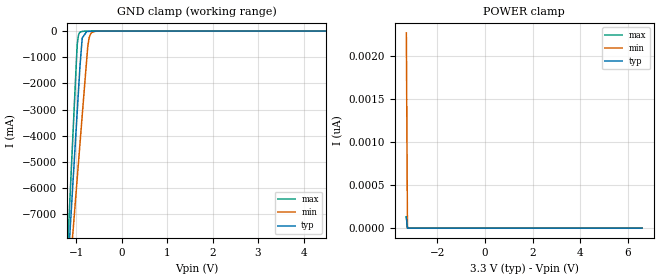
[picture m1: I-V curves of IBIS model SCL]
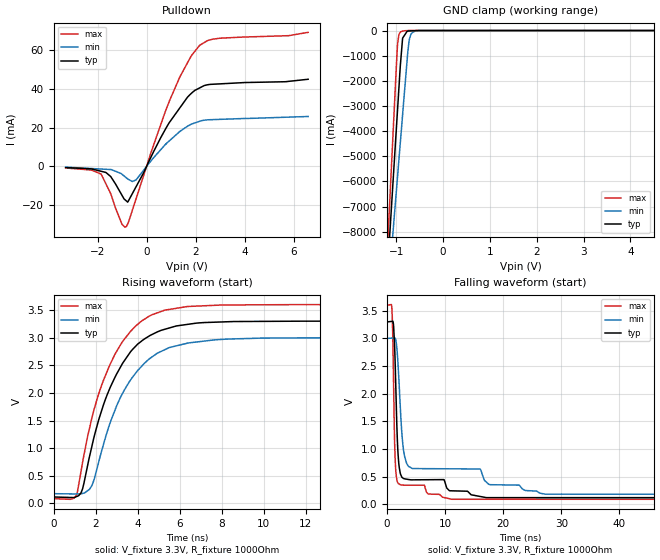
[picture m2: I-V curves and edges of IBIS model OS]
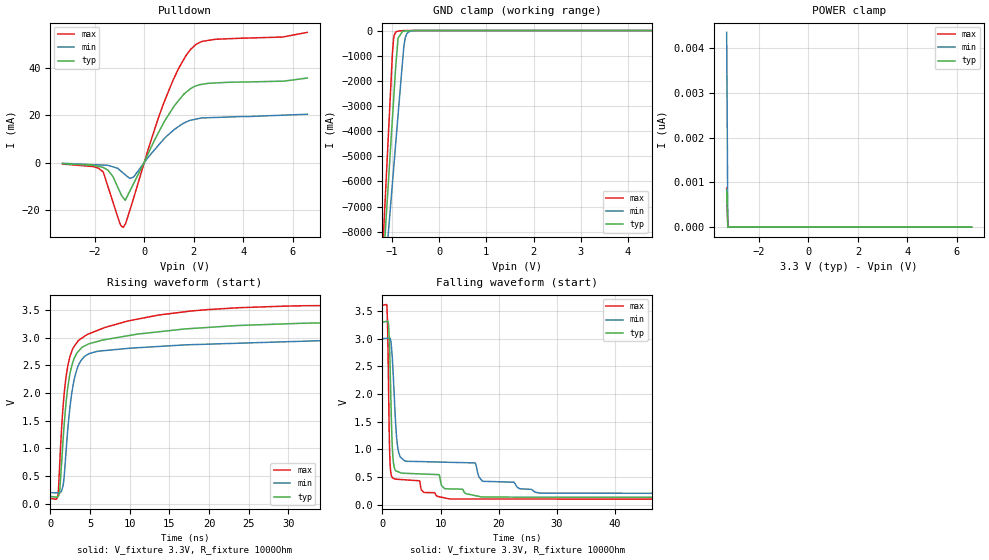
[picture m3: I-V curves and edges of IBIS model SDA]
| Texas Instruments Incorporated
| Low-Noise Clock Jitter Cleaner with Dual Loop PLLs
| Marketing part#   Voltage Range   Package-type   #pins/pkg drawing
| LM95245D   3.0V - 3.6V   SOIC   8-pin D
| LM95245DGK   3.0V - 3.6V   VSSOP   8-pin DGK
[IBIS Ver]   4.1
[File name]   lm95245.ibs
[File Rev]   1.0
[Date]   01/16/2015
[Source]   Model built from spectre simulations at:
   Texas Instruments Incorporated.
   Analog-eLab, HPA
   12500 TI Blvd
   Dallas, TX -75243
   For Support e-mail: elab_ibis@list.ti.com
[Notes]   Revision History
   Rev 1.0: 01/16/2015
   - Leakage currents at limits are high due to reverse conduction through ESD cell when reversed biased
   - Pulldown non-monotonic
   - ccomp values are based on PVT settings:
   MIN: Low Voltage, High Temperature, Weak Process
   TYP: Nominal Voltage, Nominal Temperature, Nominal Process
   MAX: High Voltage, Low Temperature, Fast Process
   - C_comp although listed in numerical order of value are obtained from varying PVT conditions.
   For PVT conditions for each specific value, refer to the buffer description under respective [Model].
   IBIS model user is responsible for using appropriate C_comp to simulate for Signal Integrity.
[Disclaimer]  This model is designed as an aid for customers of Texas Instruments
 TI and its licensors and suppliers make no warranties, either expressed
 or implied, with respect to this  model, including the warranties of
 merchantability or fitness for a particular purpose.
 The model is provided solely on an "as is" basis. The entire risk as to
 its quality and performance is with the customer.
[Copyright] (C)Copyright 2015 Texas Instruments Incorporated.
   All rights reserved.
[Component]   LM95245D
[Manufacturer]  Texas Instruments Incorporated
[Package]   |8-pin SOIC D package
|   typ   min   max
R_pkg   0.05625   0.05284   0.06331
L_pkg   2.58853nH   2.31916nH   3.13433nH
C_pkg   0.38513pF   0.35622pF   0.44246pF
[Pin]   signal_name   model_name   R_pin   L_pin   C_pin
1   VDD   POWER   0.06331   3.13433nH  0.44246pF
2   D+   NC   0.05416   2.35171nH  0.35866pF
3   D-   NC   0.05284   2.31916nH  0.35622pF
4   T_CRITB   TCRIT   0.05744   2.97557nH  0.43337pF
5   GND   GND   0.02710   2.35557nH  0.47000pF
6   OSB/A0   OS   0.05477   2.37482nH  0.35995pF
7   SMBDAT   SCL   0.05500   2.37562nH  0.36013pF
8   SMBCLK   SDA   0.02780   2.39503nH  0.47300pF
[Component]   LM95245DGK
[Manufacturer]  Texas Instruments Incorporated
[Package]   |8-pin VSSOP DGK package
|   typ   min   max
R_pkg   0.0511   0.0264   0.0795
L_pkg   1.4234n   1.2768n   1.6654n
C_pkg   0.4076p   0.3718p   0.4371p
[Pin]   signal_name   model_name   R_pin   L_pin   C_pin
1   VDD   POWER   0.04246  1.34504n  0.39979p
2   D+   NC   0.07486  1.58742n  0.39064p
3   D-   NC   0.07239  1.55295n  0.38849p
4   T_CRITB   TCRIT   0.07953  1.66542n  0.37176p
5   GND   GND   0.03169  1.33577n  0.42282p
6   OSB/A0   OS   0.04074  1.27734n  0.42502p
7   SMBDAT   SCL   0.04076  1.27679n  0.42518p
8   SMBCLK   SDA   0.02644  1.34611n  0.43708p
| Models and submodels in the file (4): SCL (Input), OS (I/O_open_drain), SDA (I/O_open_drain), TCRIT (Open_drain)
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|   Model SCL
[Model]   SCL
Model_type   Input
Vinl = .8
Vinh = 2
|   typ   min   max
|   (nom PVT)   (fast PVT)   (slow PVT)
| Where   nom PVT is  Nominal Process, 3.3V, 27C
|   Fast PVT is Strong Process, 3.6V, -40C
|   Slow PVT is Weak Process, 3.0V, 125C
C_comp   0.3623p   0.3293p   0.3941p
[Voltage Range]   3.3   3   3.6
[Temperature Range]   27   125   -40
[Power Clamp Reference]   3.3   3   3.6
[GND Clamp Reference]   0   0   0
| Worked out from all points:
|   GND clamp passes 1 mA (typ) near -0.57 V on its own axis
[GND Clamp]
|   Voltage   I(typ)   I(min)   I(max)
-3.3V     -70.34A    -56.69A    -86.62A
-1.259V   -11.24A    -11.81A    -10.92A
-1.065V   -5.628A    -7.559A    -3.742A
-974.5mV  -3.016A    -5.576A    -480.3mA
-949.7mV  -2.303A    -5.034A    -160.9mA
-900.2mV  -991.5mA   -3.951A    -28.18mA
-867.1mV  -266.8mA   -3.227A    -14.21mA
-747.5mV  -12.69mA   -642.4mA   -1.498mA
-722.7mV  -11.02mA   -323.9mA   -963.1uA
-685.6mV  -8.52mA    -119.6mA   -418.1uA
-599mV    -2.676mA   -14.83mA   -69.82uA
6.59V     0A         0A         0A
[POWER Clamp]
|   Voltage   I(typ)   I(min)   I(max)
-3.3V     131.5pA    2.275nA    131.1pA
-3.254V   1.158pA    0A         2.256pA
-3.253V   0A         0A         0A
6.59V     0A         0A         0A
|   Model OAB/A0
[Model]   OS
Model_type   I/O_open_drain
Polarity   Inverting
Enable   Active-Low
Vinl = .8
Vinh = 2
Vmeas = 1.65
Vref = 1.65
Cref = 15pF
Rref = 1000
|   typ   min   max
|   (nom PVT)   (fast PVT)   (slow PVT)
| Where   nom PVT is  Nominal Process, 3.3V, 27C
|   Fast PVT is Strong Process, 3.6V, -40C
|   Slow PVT is Weak Process, 3.0V, 125C
C_comp   0.9208p   0.8997p   0.9357p
|C_comp (ON state)   0.9208p   0.8997p   0.9357p
|C_comp (OFF state)   0.9379p   0.8833p   0.9766p
[Voltage Range]   3.3   3   3.6
[Temperature Range]   27   125   -40
[Pullup Reference]   3.3   3   3.6
[Pulldown Reference]   0   0   0
[Power Clamp Reference]   3.3   3   3.6
[GND Clamp Reference]   0   0   0
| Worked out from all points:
|   slope of the pulldown table from 0 to 0.495 V, typ, clamps not added: 38.7 ohm
|   GND clamp passes 1 mA (typ) near -0.58 V on its own axis
|   falling waveform, V_fixture 3.3V, R_fixture 1000Ohm: 20-80 % time 642ps typ, 1.42ns min, 399ps max; typ from 3.3 V to 0.117 V
|   rising waveform, V_fixture 3.3V, R_fixture 1000Ohm: 20-80 % time 1.86ns typ, 1.93ns min, 1.83ns max; typ from 0.117 V to 3.3 V
[Pulldown]
|   Voltage   I(typ)   I(min)   I(max)
-3.3V     -602.7uA   -366.2uA   -793.4uA
-1.853V   -2.501mA   -1.35mA    -3.94mA
-1.461V   -5.231mA   -1.616mA   -14.08mA
-1.012V   -14.69mA   -3.933mA   -29.57mA
-856.9mV  -17.46mA   -5.538mA   -31.3mA
-768.1mV  -18.44mA   -6.46mA    -29.66mA
-433mV    -10.6mA    -6.983mA   -16.91mA
949.5mV   23.01mA    13.43mA    34.32mA
1.803V    37.43mA    21.67mA    56.62mA
2.152V    40.44mA    23.24mA    62.29mA
2.988V    42.62mA    24.3mA     66.19mA
6.59V     45mA       25.78mA    69.23mA
[GND Clamp]
|   Voltage   I(typ)   I(min)   I(max)
-3.3V     -72.96A    -59.34A    -89.27A
-1.237V   -10.98A    -11.8A     -10.43A
-1.065V   -5.822A    -7.852A    -3.87A
-974.5mV  -3.128A    -5.788A    -530.7mA
-949.7mV  -2.396A    -5.225A    -195.9mA
-900.2mV  -1.047A    -4.1A      -44.21mA
-867.1mV  -303.4mA   -3.348A    -23.16mA
-754.8mV  -22.12mA   -833.3mA   -2.647mA
-730mV    -19.18mA   -431.7mA   -1.412mA
-680.5mV  -13.31mA   -127.3mA   -515.4uA
-606.3mV  -4.498mA   -27.6mA    -93.13uA
6.59V     0A         0A         0A
[Ramp]
R_load = 1000
|   typ   min   max
dV/dt_r   1.90954/1.8473e-09   1.69358/1.93096e-09   2.10714/1.82203e-09
dV/dt_f   1.90954/6.42261e-10   1.6936/1.41537e-09   2.10727/3.95718e-10
[Falling Waveform]
V_fixture = 3.3V
V_fixture_min = 3V
V_fixture_max = 3.6V
R_fixture = 1000Ohm
C_fixture = 0F
|   Time   V(typ)   V(min)   V(max)
0s        3.3V       3V         3.6V
823ps     3.309V     3.007V     3.569V
1.13ns    3.232V     3.01V      2.174V
1.51ns    2.127V     2.97V      601.6mV
1.908ns   892.3mV    2.509V     379.4mV
2.411ns   522.6mV    1.513V     346.5mV
3.005ns   459.6mV    874mV      345mV
4.324ns   440.8mV    647.6mV    344.4mV
27.3ns    118.2mV    180.9mV    88.98mV
100ns     117.4mV    177.3mV    87.88mV
[Rising Waveform]
V_fixture = 3.3V
V_fixture_min = 3V
V_fixture_max = 3.6V
R_fixture = 1000Ohm
C_fixture = 0F
|   Time   V(typ)   V(min)   V(max)
0s        117.4mV    177.3mV    87.86mV
969.5ps   108.3mV    172.6mV    94.41mV
1.108ns   126.9mV    171.9mV    172mV
1.31ns    193.9mV    174.8mV    584.4mV
1.836ns   1.052V     331.3mV    1.562V
2.138ns   1.497V     731.9mV    1.97V
3.262ns   2.519V     1.976V     2.917V
4.574ns   3.035V     2.621V     3.393V
6.346ns   3.239V     2.898V     3.562V
100ns     3.3V       3V         3.6V
|   Model SDA
[Model]   SDA
Model_type   I/O_open_drain
Polarity   Inverting
Enable   Active-Low
Vinl = .8
Vinh = 2
Vmeas = 1.65
Vref = 1.65
Cref = 15pF
Rref = 1000
|   typ   min   max
|   (nom PVT)   (fast PVT)   (slow PVT)
| Where   nom PVT is  Nominal Process, 3.3V, 27C
|   Fast PVT is Strong Process, 3.6V, -40C
|   Slow PVT is Weak Process, 3.0V, 125C
C_comp   0.8159p   0.7677p   0.8516p
|C_comp (ON state)   0.8159p   0.7677p   0.8516p
|C_comp (OFF state)   0.8244p   0.7598p   0.8719p
[Voltage Range]   3.3   3   3.6
[Temperature Range]   27   125   -40
[Pullup Reference]   3.3   3   3.6
[Pulldown Reference]   0   0   0
[Power Clamp Reference]   3.3   3   3.6
[GND Clamp Reference]   0   0   0
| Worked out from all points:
|   slope of the pulldown table from 0 to 0.495 V, typ, clamps not added: 45.3 ohm
|   GND clamp passes 1 mA (typ) near -0.55 V on its own axis
|   falling waveform, V_fixture 3.3V, R_fixture 1000Ohm: 20-80 % time 617ps typ, 12ns min, 351ps max; typ from 3.3 V to 0.134 V
|   rising waveform, V_fixture 3.3V, R_fixture 1000Ohm: 20-80 % time 1.71ns typ, 1.49ns min, 2.08ns max; typ from 0.134 V to 3.3 V
[Pulldown]
|   Voltage   I(typ)   I(min)   I(max)
-3.3V     -460.1uA   -284.7uA   -598.1uA
-1.655V   -2.053mA   -1.055mA   -3.941mA
-1.263V   -5.86mA    -1.798mA   -16.61mA
-986.8mV  -12.22mA   -3.164mA   -25.47mA
-838.3mV  -14.93mA   -4.498mA   -27.19mA
-768.1mV  -15.9mA    -5.128mA   -25.94mA
-425.7mV  -8.763mA   -6.038mA   -14.89mA
776.1mV   16.56mA    9.733mA    24.73mA
1.37V     25.89mA    15.06mA    39.22mA
1.896V    31.3mA     17.88mA    47.92mA
2.882V    33.55mA    19.01mA    51.94mA
6.59V     35.61mA    20.37mA    54.87mA
[GND Clamp]
|   Voltage   I(typ)   I(min)   I(max)
-3.3V     -72.96A    -59.34A    -89.27A
-1.263V   -11.74A    -12.39A    -11.41A
-1.111V   -7.182A    -8.894A    -5.597A
-1.065V   -5.821A    -7.851A    -3.869A
-986.8mV  -3.495A    -6.069A    -910.3mA
-949.7mV  -2.395A    -5.224A    -195.9mA
-887.8mV  -768.9mA   -3.814A    -33.21mA
-867.1mV  -302.9mA   -3.343A    -24.81mA
-747.5mV  -21.85mA   -684.3mA   -1.579mA
-722.7mV  -19.25mA   -356.9mA   -1.438mA
-599mV    -6.264mA   -23.95mA   -510.6uA
6.59V     0A         0A         0A
[POWER Clamp]
|   Voltage   I(typ)   I(min)   I(max)
-3.3V     844.3pA    4.355nA    876.3pA
-3.254V   7.436pA    0A         15.08pA
-3.253V   0A         0A         0A
6.59V     0A         0A         0A
[Ramp]
R_load = 1000
|   typ   min   max
dV/dt_r   1.89964/1.68373e-09   1.6776/1.48622e-09   2.10017/2.02042e-09
dV/dt_f   1.8997/6.16992e-10   1.6784/8.06083e-09   2.10018/3.50292e-10
[Falling Waveform]
V_fixture = 3.3V
V_fixture_min = 3V
V_fixture_max = 3.6V
R_fixture = 1000Ohm
C_fixture = 0F
|   Time   V(typ)   V(min)   V(max)
0s        3.3V       3V         3.6V
813.3ps   3.312V     3.007V     3.527V
1.219ns   2.902V     3.01V      1.095V
1.517ns   1.685V     2.906V     541.4mV
1.946ns   732.1mV    2.185V     475.3mV
2.332ns   612.5mV    1.382V     463.3mV
2.814ns   593.1mV    941.5mV    459.9mV
7.149ns   555.8mV    779.2mV    225.2mV
27.24ns   139.5mV    211.3mV    105.1mV
100ns     133.8mV    202.7mV    99.7mV
[Rising Waveform]
V_fixture = 3.3V
V_fixture_min = 3V
V_fixture_max = 3.6V
R_fixture = 1000Ohm
C_fixture = 0F
|   Time   V(typ)   V(min)   V(max)
0s        133.8mV    202.6mV    99.7mV
959.3ps   130.2mV    198.2mV    151.2mV
1.186ns   219.1mV    197.2mV    710.1mV
1.603ns   1.124V     319.2mV    1.738V
2.16ns    2.05V      1.265V     2.449V
2.788ns   2.532V     2.066V     2.788V
4.386ns   2.856V     2.67V      3.033V
9.628ns   3.032V     2.805V     3.297V
29.77ns   3.251V     2.928V     3.571V
100ns     3.3V       2.999V     3.6V
